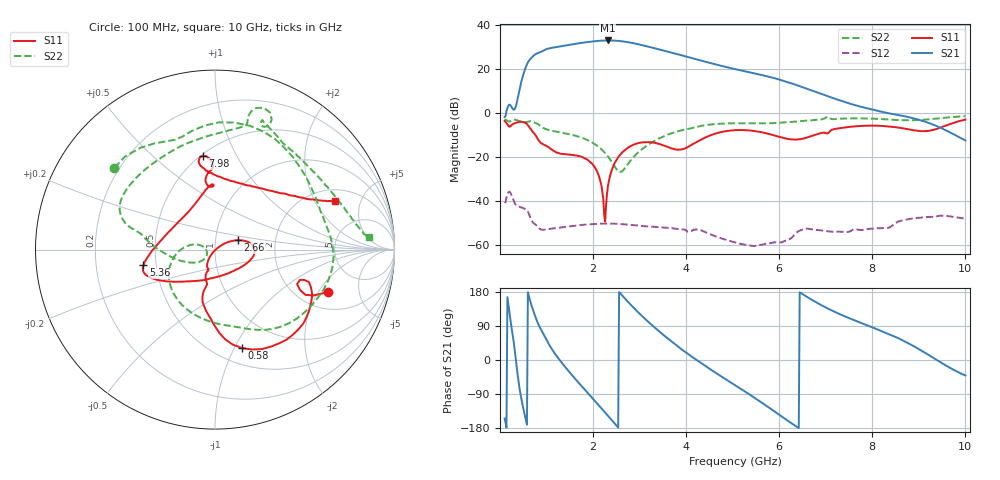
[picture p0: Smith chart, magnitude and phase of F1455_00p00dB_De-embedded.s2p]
! Integrated Device Technology
! Corporate Headquarters
! 6024 Silver Creek Valley Road
! San Jose, CA 95138  USA
! Phone:  1-408-284-8200
! Toll Free:  1-800-223-1366
! Webpage:  http://www.idt.com/
! Timing and RF Division
! 515 Groton Road, Suite 102
! Westford, MA 01886-6024
! Device:  F1455
! Description: 6-bit 0.5 dB Transmit Variable Gain Amplifier
! Frequency:  1400.0 -  2300.00 MHz
! Package:  6x6 mm Thin QFN Plastic Package: 28 pin
! State:  0
! Atten State:  0.0 dB
! Voltage:  +5.00 Volts
! Current:  213.756 mA
! Data:  The device was measured on a the F1455 evaluation board which has
!  individual transmission lines to the RF pins.  Data was collected
!  using a calibrated network analyzer.  The evaluation board was
!  de-embedded using a TRL calibration technique.
!  The reference plane is the edge of the package pin.
!  Pin  1 = CSb
!  Pin  2 = DATA
!  Pin  3 = CLK
!  Pin  4 = RSET
!  Pin  5 = GND
!  Pin  6 = RFIN  = Port 1
!  Pin  7 = GND
!  Pin  8 = NC
!  Pin  9 = NC
!  Pin 10 = NC
!  Pin 11 = NC
!  Pin 12 = NC
!  Pin 13 = NC
!  Pin 14 = /STBY
!  Pin 15 = GND
!  Pin 16 = RFOUT  = Port 2
!  Pin 17 = GND
!  Pin 18 = NC
!  Pin 19 = NC
!  Pin 20 = NC
!  Pin 21 = GND
!  Pin 22 = NC
!  Pin 23 = GND
!  Pin 24 = NC
!  Pin 25 = NC
!  Pin 26 = NC
!  Pin 27 = GND
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# GHz S dB R 50
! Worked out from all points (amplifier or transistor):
!   496 points, 100 MHz to 10 GHz, reference 50 ohm
!   highest |S21| = 33.1 dB at 2.32 GHz (marker M1)
!   |S21| within 3 dB of that: 1.208 GHz to 3.223 GHz (2.015 GHz wide, 91 % of centre)
!   unconditionally stable (mu >= 1): start of sweep to end of sweep
!   at 1.74 GHz: K = 4.02, MAG = 32.4 dB, |S12| = -50.8 dB
!   at 5.06 GHz: K = 23.03, MAG = 22.7 dB, |S12| = -58.7 dB
!   at 10 GHz: K = 62.68, MAG = -3.2 dB, |S12| = -47.9 dB
!   S11 on the Smith chart (normalised r, x): 100 MHz: 2.83, -2.43; 580 MHz: 0.66, -1.07; 2.66 GHz: 1.29, +0.14; 5.36 GHz: 0.42, -0.09; 7.98 GHz: 0.51, +0.74; 10 GHz: 2.60, +2.95
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0.1  -3.47 -20.6  -1.67 -154.6  -40.72 39.0  -2.83 140.8
0.4  -3.96 -36.5  8.79 -57.7  -42.33 -109.4  -3.41 50.3
0.58  -4.89 -74.6  22.28 -170.7  -44.08 -171.2  -3.95 11.8
0.68  -7.78 -91.6  25.33 143.3  -48.71 157.4  -3.68 -14.7
0.78  -10.45 -103.3  27.08 107.8  -50.77 143.6  -4.49 -40.2
0.98  -14.57 -104.3  29.02 57.8  -52.80 123.4  -7.11 -76.2
1.14  -16.90 -110.3  29.85 24.2  -52.30 103.4  -8.02 -96.5
1.34  -18.42 -108.1  30.61 -9.1  -51.77 82.1  -8.83 -118.9
1.76  -19.81 -115.8  32.03 -69.6  -50.69 48.3  -11.08 -156.2
2.04  -24.65 -124.0  32.77 -108.1  -50.26 29.8  -14.02 -178.0
2.32  -33.04 33.3  33.11 -147.2  -50.07 12.3  -19.60 164.2
2.66  -17.13 22.0  32.64 165.6  -50.40 -6.7  -25.53 -148.0
3  -13.42 5.6  31.26 122.3  -51.06 -22.2  -17.21 -148.1
3.4  -13.77 -16.8  29.17 77.7  -51.69 -36.9  -11.66 -172.9
3.98  -15.89 -96.2  25.88 21.2  -53.02 -60.4  -7.38 167.7
4.5  -10.17 -145.0  22.96 -23.0  -54.71 -83.8  -5.14 160.5
5.06  -7.64 -161.4  20.05 -67.2  -58.68 -88.5  -4.50 148.1
5.36  -7.79 -167.8  18.65 -90.8  -59.96 -83.6  -4.52 137.7
6.7  -10.26 105.2  10.42 158.9  -52.65 -119.9  -3.13 78.0
7.98  -5.58 97.3  1.79 87.1  -52.37 -173.4  -2.39 68.7
8.36  -5.97 100.4  -0.01 68.2  -51.89 -175.0  -2.79 62.2
10  -2.84 22.2  -12.32 -40.8  -47.93 95.4  -1.28 4.5
